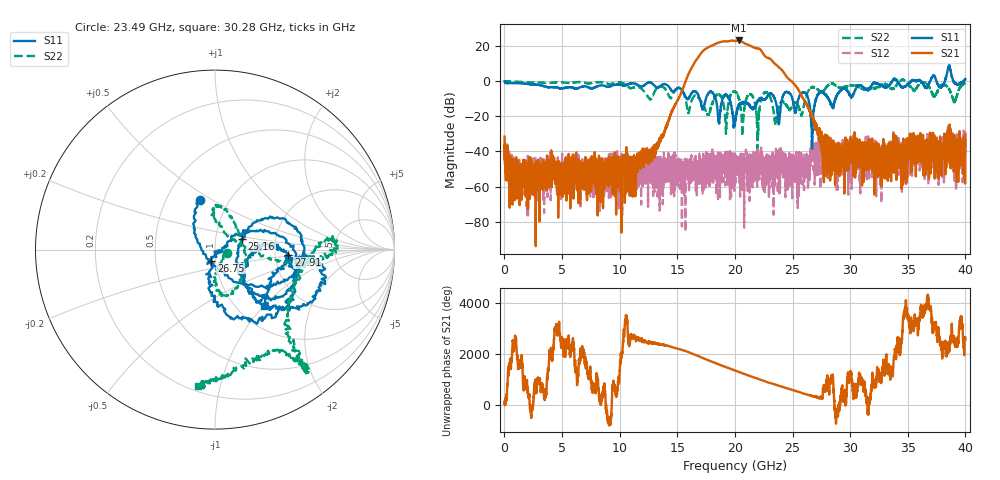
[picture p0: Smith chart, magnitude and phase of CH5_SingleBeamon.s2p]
!Keysight Technologies,N5245B,MY57181321,A.14.80.03
!Date: Thursday, March 28, 2024 18:51:33
!Correction: S11(C  2-Port  )
!S21(C  2-Port  )
!S12(C  2-Port  )
!S22(C  2-Port  )
!S2P File: Measurements: S11, S21, S12, S22:
# Hz S  RI  R 50
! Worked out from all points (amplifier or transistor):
!   4000 points, 10 MHz to 40 GHz, reference 50 ohm
!   highest |S21| = 23.1 dB at 20.33 GHz (marker M1)
!   |S21| within 3 dB of that: 17.97 GHz to 21.33 GHz (3.353 GHz wide, 17.1 % of centre)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
!   unconditionally stable (mu >= 1): 15.92 MHz to 33.64 GHz; 36.12 GHz to 36.93 GHz; 38.95 GHz to 39.87 GHz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
!   at 6.67 GHz: K = 2090.83, MAG = -34.8 dB, |S12| = -49.7 dB
!   at 20.01 GHz: K = 7.31, MAG = 24.1 dB, |S12| = -48.6 dB
!   at 40 GHz: K = -60.36, MSG = 0.2 dB, |S12| = -30.5 dB
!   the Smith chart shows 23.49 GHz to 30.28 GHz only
!   S11 on the Smith chart (normalised r, x): 23.49 GHz: 0.73, +0.45; 25.16 GHz: 1.34, +0.17; 26.75 GHz: 0.95, -0.12; 27.91 GHz: 2.38, -0.16; 30.28 GHz: 1.33, -1.00
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1e7  0.9982 -0.0418  -0.0175 0.0199  0.00373 -0.00203  -0.9694 0.0564
6.68e9  0.5043 0.4674  -0.00314 -0.00102  -0.0014 0.0018  0.9297 0.0917
1.334e10  -0.6007 -0.282  -0.011 -0.0109  0.000141 -0.000975  -0.6819 -0.0648
1.706e10  0.19 0.1301  2.038 5.857  -0.0025 -0.000284  0.1067 0.237
1.752e10  0.2544 -0.228  8.072 -2.685  -0.000137 0.00217  -0.1161 0.0585
1.797e10  0.4653 -0.1506  -1.66 -10.02  0.00161 -0.00256  0.0521 -0.1927
1.847e10  0.1745 0.0226  -12.01 1.77  0.00164 -0.00344  0.3947 -0.1475
1.897e10  -0.0564 -0.3273  1.444 13.38  -0.00513 0.00232  0.2559 0.0125
1.949e10  0.1978 -0.2473  13.62 -1.166  3.82e-05 0.00289  -0.2022 -0.1916
2.001e10  -0.0463 0.0447  -0.9756 -13.9  0.00214 0.00302  -0.2291 -0.4375
2.033e10  -0.1909 -0.104  -12.29 -7.412  0.000429 0.00702  -0.0743 -0.3105
2.098e10  0.2206 -0.0907  -1.82 11.2  -0.00332 -0.00294  -0.1419 0.2817
2.153e10  -0.0604 0.1571  9.073 2.692  -0.000841 0.000461  -0.3078 0.2051
2.209e10  -0.1701 -0.2487  2.16 -8.079  0.00743 4.76e-05  0.1477 0.0032
2.349e10  -0.0815 0.279  0.6948 2.992  -0.00456 -0.00198  0.0653 -0.0213
2.516e10  0.1499 0.0608  -0.7611 -0.2759  0.00075 0.00221  0.0413 0.2357
2.667e10  0.0402 -0.0115  0.0972 -0.0136  0.000957 0.0086  0.6449 -0.00513
2.675e10  -0.0205 -0.0612  0.0902 -0.0444  0.00899 -0.0087  0.6832 0.023
2.791e10  0.4091 -0.0285  -0.00934 -0.00256  0.00441 0.0062  0.4111 -0.5103
3.028e10  0.2753 -0.3122  0.00928 -0.00792  0.00544 -0.00232  -0.0953 -0.7604
3.334e10  0.1652 -0.7233  0.00158 -0.00103  -0.00103 -0.0117  -0.3531 -0.6287
4e10  -0.8562 -0.7684  0.0247 0.0188  0.0286 0.0087  0.4986 0.6334
